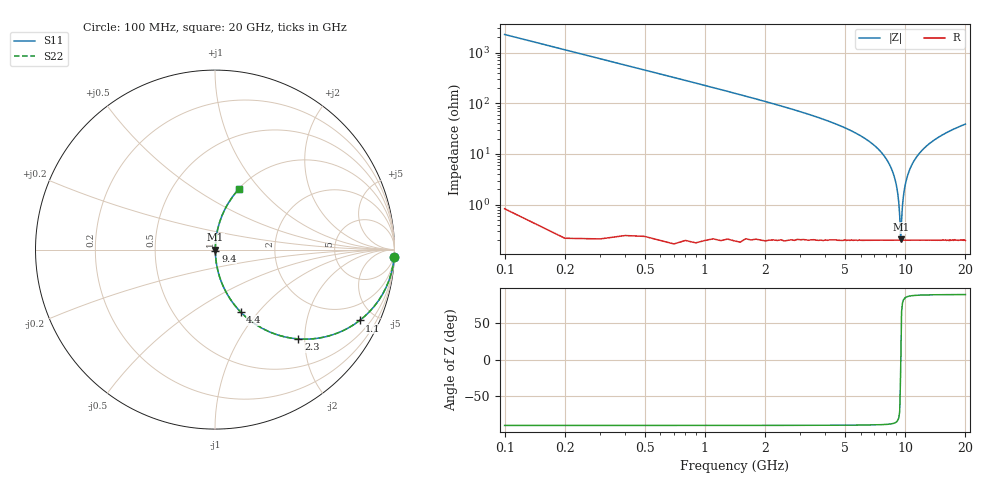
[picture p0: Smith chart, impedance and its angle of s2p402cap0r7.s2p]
! AVX Thin Film Operation		Date: April 2003
! Description: Accu-P® Series, Thin Film, SMD, RF Capacitor
! Part Number: 04021J0R7ABS
! 50 MHz  -  20 GHz
! Serial Measurements
# hz S db R 50
!	S11		S21		S12		S22
!	dB	Phase	dB	Phase	dB	Phase	dB	Phase
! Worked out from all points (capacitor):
!   200 points, 100 MHz to 20 GHz, reference 50 ohm
!   read as one part in series: C = 700 fF near 200 MHz
!   lowest |Z| = 208 mohm at 9.5 GHz (marker M1)
!   series resonance near 9.511 GHz, so ESL is about 400 pH
!   S11 on the Smith chart (normalised r, x): 100 MHz: 1, -45; 1.1 GHz: 1.00, -4.08; 2.3 GHz: 1.00, -1.86; 4.4 GHz: 1.00, -0.81; 9.4 GHz: 1.00, -0.01; 20 GHz: 1.00, +0.78
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1e8  -0.01 -2.5  -27.14 87.5  -27.14 87.5  -0.01 -2.5
2e8  -0.03 -5.0  -21.14 85.0  -21.14 85.0  -0.03 -5.0
4e8  -0.13 -10.0  -15.21 80.0  -15.21 80.0  -0.13 -10.0
7e8  -0.40 -17.2  -10.58 72.8  -10.58 72.8  -0.40 -17.2
1.1e9  -0.94 -26.1  -7.13 63.8  -7.13 63.8  -0.94 -26.1
2.3e9  -3.34 -47.0  -2.72 42.9  -2.72 42.9  -3.34 -47.0
3.5e9  -6.21 -60.5  -1.20 29.3  -1.20 29.3  -6.21 -60.5
4.4e9  -8.50 -67.7  -0.68 22.1  -0.68 22.1  -8.50 -67.7
6.8e9  -15.86 -80.0  -0.13 9.3  -0.13 9.3  -15.86 -80.0
7.9e9  -21.04 -83.6  -0.05 5.1  -0.05 5.1  -21.04 -83.6
8.7e9  -27.41 -84.9  -0.03 2.4  -0.03 2.4  -27.41 -84.9
9.2e9  -35.91 -81.9  -0.02 0.9  -0.02 0.9  -35.91 -81.9
9.4e9  -44.49 -70.1  -0.02 0.3  -0.02 0.3  -44.49 -70.1
9.5e9  -53.66 -15.9  -0.02 0.0  -0.02 0.0  -53.66 -15.9
9.7e9  -40.37 77.4  -0.02 -0.5  -0.02 -0.5  -40.37 77.4
9.9e9  -34.33 82.9  -0.02 -1.1  -0.02 -1.1  -34.33 82.9
1.01e10  -30.83 84.4  -0.02 -1.6  -0.02 -1.6  -30.83 84.4
1.06e10  -25.72 84.8  -0.03 -3.0  -0.03 -3.0  -25.72 84.8
1.13e10  -21.68 83.9  -0.05 -4.7  -0.05 -4.7  -21.68 83.9
1.34e10  -15.68 79.8  -0.14 -9.5  -0.14 -9.5  -15.68 79.8
1.67e10  -11.30 73.8  -0.35 -15.8  -0.35 -15.8  -11.30 73.8
2e10  -8.83 68.5  -0.63 -21.2  -0.63 -21.2  -8.83 68.5
